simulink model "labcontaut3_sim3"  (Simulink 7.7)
settings: Solver=ode45  StartTime=0.0  StopTime=10.0  RelTol=1e-3
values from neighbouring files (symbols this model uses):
  F = tf(10^2*zpk([],[-10 -10],1))    [labcontaut3.m]

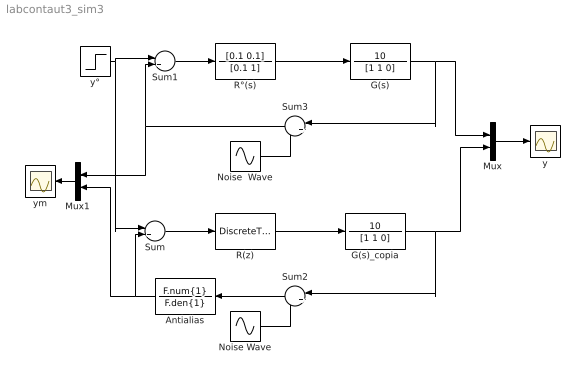
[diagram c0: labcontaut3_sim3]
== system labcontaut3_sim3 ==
  Antialias : TransferFcn  Numerator=F.num{1}  Denominator=F.den{1}
  G(s) : TransferFcn  Numerator=10  Denominator=[1 1 0]
  G(s)_copia : TransferFcn  Numerator=10  Denominator=[1 1 0]
  Mux : Mux  Inputs=2
  Mux1 : Mux  Inputs=2
  Noise  Wave : Sin  Amplitude=0.05  Frequency=500  SampleTime=0
  Noise Wave : Sin  Amplitude=0.05  Frequency=500  SampleTime=0
  R(z) : DiscreteTransferFcn  Numerator=[1.1 -1]  Denominator=[2 -1]  SampleTime=0.1
  R°(s) : TransferFcn  Numerator=[0.1 0.1]  Denominator=[0.1 1]
  Sum : Sum  Inputs=|+-
  Sum1 : Sum  Inputs=|+-
  Sum2 : Sum  Inputs=|++
  Sum3 : Sum  Inputs=|++
  y : Scope
  ym : Scope
  y° : Step  Time=0  SampleTime=0
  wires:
  Sum1/1 -> R°(s)/1
  y°/1 -> Sum1/1, Sum/1
  G(s)/1 -> Mux/1, Sum3/1
  Mux/1 -> y/1
  R°(s)/1 -> G(s)/1
  Sum/1 -> R(z)/1
  G(s)_copia/1 -> Mux/2, Sum2/1
  R(z)/1 -> G(s)_copia/1
  Sum2/1 -> Antialias/1
  Noise Wave/1 -> Sum2/2
  Sum3/1 -> Sum1/2, Mux1/1
  Noise  Wave/1 -> Sum3/2
  Mux1/1 -> ym/1
  Antialias/1 -> Sum/2, Mux1/2
